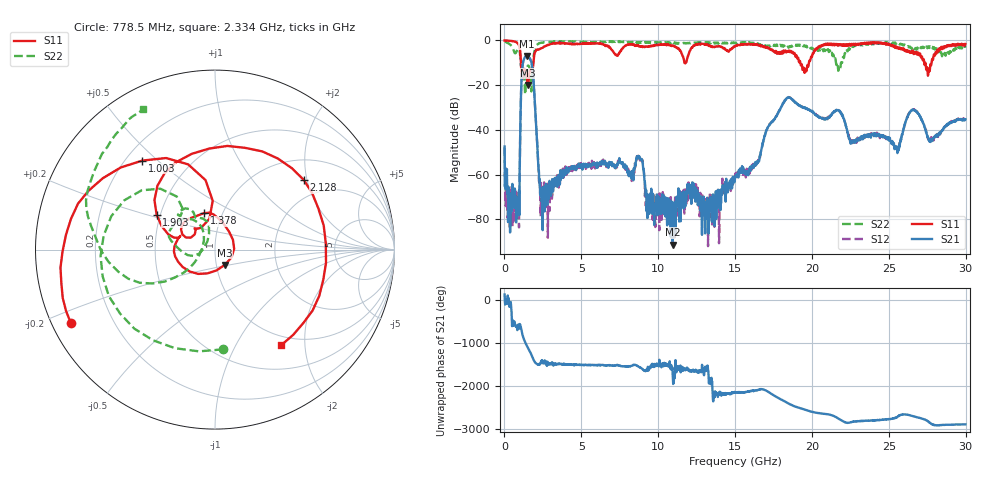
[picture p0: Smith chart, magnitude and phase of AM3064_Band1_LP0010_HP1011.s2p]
# Hz S DB R 50.0
!freq dBS11 angS11 dBS21 angS21 dBS12 angS12 dBS22 angS22
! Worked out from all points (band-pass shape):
!   1600 points, 10 MHz to 29.98 GHz, reference 50 ohm
!   highest |S21| = -6.99 dB at 1.453 GHz (marker M1); lowest = -91.3 dB at 10.94 GHz (marker M2)
!   |S21| within 3 dB of the highest: 1.204 GHz to 1.757 GHz (553 MHz wide, 37.3 % of centre)
!   lowest |S11| = -19.9 dB at 1.547 GHz (marker M3), VSWR 1.23, Z = 55 - j9.45 ohm
!   |S11| at or under -10 dB: 1.071 GHz to 1.881 GHz (810.8 MHz wide, 54.9 % of centre); 19.24 GHz to 19.81 GHz (562.7 MHz wide, 2.88 % of centre); 27.38 GHz to 27.78 GHz (405 MHz wide, 1.47 % of centre)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
!   |S22| runs from -24.1 to -0.3 dB; largest |S21 - S12| = 0.0054
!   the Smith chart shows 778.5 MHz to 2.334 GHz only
!   S11 on the Smith chart (normalised r, x): 778.5 MHz: 0.05, -0.24; 1.003 GHz: 0.27, +0.45; 1.378 GHz: 0.82, +0.35; 1.903 GHz: 0.48, +0.22; 2.128 GHz: 1.49, +1.91; 2.334 GHz: 0.85, -1.56
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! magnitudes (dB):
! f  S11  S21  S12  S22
! 10 MHz  0.0  -47.4  -47.9  -0.3
! 328.6 MHz  -0.2  -79.0  -68.9  -1.6
! 778.5 MHz  -0.9  -73.6  -73.5  -5.1
! 1.003 GHz  -3.9  -51.3  -51.0  -5.6
! 1.172 GHz  -16.3  -11.5  -11.4  -12.4
! 1.378 GHz  -13.5  -7.1  -7.2  -20.8
! 1.453 GHz  -16.5  -7.0  -6.9  -13.7
! 1.547 GHz  -19.9  -7.3  -7.3  -11.3
! 1.903 GHz  -8.4  -19.3  -19.2  -6.8
! 2.128 GHz  -4.0  -45.7  -45.5  -1.9
! 2.334 GHz  -3.8  -69.0  -70.6  -1.1
! 5.015 GHz  -1.5  -56.9  -55.6  -0.7
! 8.763 GHz  -2.6  -52.7  -52.2  -1.1
! 9.344 GHz  -2.8  -70.7  -70.5  -1.0
! 10 GHz  -2.0  -69.6  -70.7  -0.9
! 10.94 GHz  -2.4  -91.3  -72.8  -1.2
! 15 GHz  -2.7  -61.7  -61.1  -1.2
! 18.34 GHz  -5.3  -25.9  -25.8  -2.7
! 19.99 GHz  -7.4  -31.7  -31.8  -3.4
! 25 GHz  -1.5  -43.3  -43.4  -1.2
! 27.56 GHz  -15.2  -43.5  -44.3  -2.8
! 29.98 GHz  -1.6  -35.3  -35.6  -3.2
